(* Logix 5000 AddOnInstructionDefinition export NTEC_READ; software revision ? *)

TYPE NTEC_Axis :   // NTEC Axis:
STRUCT
   StatDriveCommsOK : BOOL;   // Drive is communicating over ENET IP
   StatServoActionStatus : BOOL;   // Motion is enabled and holding position under power.
   StatDriveWarning : BOOL;   // Drive has a Warning
   StatDriveFault : BOOL;   // Drive is Faulted
   StatMotion_AtTarget : BOOL;   // Motion Target Reached
   StatMotion_FollowingError : BOOL;   // Following Error Fault
   StatMotion_LimitExceeded : BOOL;   // Speed or Position Limit Exceeded
   StatMotion_Halt : BOOL;   // Motor is in Halt, still powered on
   StatQuckStop : BOOL;   // Motor is powered off in Quick Stop
   StatMotion_Homed : BOOL;   // Motion Coordinate System Homed
   StatNewCmdToggle : BOOL;   // Bit toggles after new command accepted
   StatCommandError : BOOL;   // Last Command has an Error
   StatCommandErrorCode : DINT;   // Command Error Code
   StatDriveFaultCode : DINT;   // Drive Fault Code
   StatDriveWarningCode : DINT;   // Drive Warning Code
   StatResettingFault : BOOL;   // In fault reset sequence
   StatReadResponse : DINT;   // Response from a Read CMD
   CMD_IP : BOOL;   // Command is In Process
   CMD_DN : BOOL;   // Command is Done
   CMD_ERR : BOOL;   // Command Error during Comms send to Drive
   PDI_CMD : NTEC_PDI_CMD;   // Commands from AOIs
   PDI_Status : NTEC_PDI_Status;   // Status from Drive out to AOIs
   DriveLimits : NTEC_LimitsInDrive;   // Limits read from Drive
END_STRUCT
END_TYPE

TYPE NTEC_LimitsInDrive :   // These are the limits read from the Drive
STRUCT
   PositionLimitMin : DINT;   // Minimum Allowed Position Target (607Bh:1)
   PositionLimitMax : DINT;   // Maximum Allowed Position Target (607Bh:2)
   SoftPositionLimitMin : DINT;   // Minimum Allowed Position (607Dh:1)
   SoftPositionLimitMax : DINT;   // Minimum Allowed Position (607Dh:2)
   VelocityLimitMin : DINT;   // Maximum Allowed Velocity Target negative direction
   VelocityLimitMax : DINT;   // Maximum Allowed Velocity Target positive direction (607Fh)
   MotorSpeedMin : DINT;   // Maximum motor speed in negative direction
   MotorSpeedMax : DINT;   // Maximum motor speed setting in positive direction (6080h)
   AccelLimitMax : DINT;   // Maximum Allowed Accel Target (60C5h)
   DecelLimitMax : DINT;   // Maximum Allowed Decel Target (60C6h)
   PositionWindowNeg : DINT;   // Position Window - negative direction for At Target (6067h)
   PositionWindowPos : DINT;   // Position Window -positive direction for At Target (+/- this value) (6067h)
   VelocityWindowNeg : DINT;   // Velocity Window - negative side for At Target (+/- this value) (606Dh)
   VelocityWindowPos : DINT;   // Velocity Window - positive side for At Target (+/- this value) (606Dh)
   TorqueMaxNegDir : DINT;   // Maximum Torque Target negative direction (0.1% of motor rated current 2031h) (6072h)
   TorqueMaxPosDir : DINT;   // Maximum Torque Target positive direction (0.1% of motor rated current 2031h) (6072h)
   CurrentMaxNegDir : DINT;   // Maximum Current Target negative direction (in 0.1% of rated setting 2031h) (6073h)
   CurrentMaxPosDir : DINT;   // Maximum Current Target positive direction (in 0.1% of rated setting 2031h) (6073h)
END_STRUCT
END_TYPE

TYPE NTEC_PDI_CMD :   // PDI Command Bytes
STRUCT
   SetValue1 : DINT;
   SetValue2 : INT;
   SetValue3 : SINT;
   CMD : SINT;
   DigitalOutputs : DINT;
   NanoJ_Input1 : DINT;
   Trig : BOOL;   // Trigger the Command
   Halt : BOOL;   // Command a HALT
   QuickStop : BOOL;   // Command a QuickStop
END_STRUCT
END_TYPE

TYPE NTEC_PDI_Status :   // PDI Status Bytes
STRUCT
   Status : INT;
   ErrorCode : INT;
   ReturnValue : DINT;
   PositionActualValue : DINT;
   VelocityActualValue : DINT;
   DigitalInputs : DINT;
   TorqueActualValue : INT;
   AnalogInput1 : INT;
   FollowingError : DINT;
   NanoJ_Output1 : DINT;
END_STRUCT
END_TYPE

ADD_ON_INSTRUCTION NTEC_READ   (* revision 1.6, vendor Third Coast Automation, Nashville, TN, ExecutePrescan, ExecuteEnableInFalse *)
// READ instruction reads the value of  one object from the Drive.  Enter the target object's index and sub-index (typically 16#xxxx hex values).
// Revision note:
// Release Aug 27, 2024, update CPS instructions LEN
// Help:
// AOI written by:
// Tim Cochran
// Third Coast Automation
// Nashville, TN
// MAS ERR_Codes:
// 2: Input parameter range error – review and fix input parameters.
// 3: Command Error response from the Drive after command sent.
// 10: Communications Failed to Drive.
// 11: Drive Fault during this AOIs command sequence.
// 12: Quick Stop triggered by software outside of this AOI.
// 13: Command Error response from the Drive.
// 14: Enable input changed to False during sequence due to Drive Fault or Offline.
VAR_IN_OUT
   NTEC_Axis : NTEC_Axis; {required}   // NTEC Axis Tag
END_VAR
VAR_INPUT
   Index : DINT; {required}   // Index
   SubIndex : DINT; {required}   // Sub-Index
END_VAR
VAR_OUTPUT
   EN : BOOL; {visible}   // Enabled
   DN : BOOL; {visible}   // Successfully Done
   Read_Value : DINT; {visible}   // Value Read from Drive
   ERR : BOOL; {visible}   // Instruction Error
   ERR_Code : DINT; {access Read Only, visible}   // Instruction Error Code
END_VAR
VAR
   State : DINT; {access None}
   Enable : BOOL; {access None}
   InputRangesOK : BOOL; {access None}
   local_SubIndex : DINT; {access None}
   local_Index : DINT; {access None}
   tmr_Verify : TIMER := (PRE := 20); {access None}
END_VAR

ROUTINE EnableInFalse   (* ladder *)
// Enable In False Routine
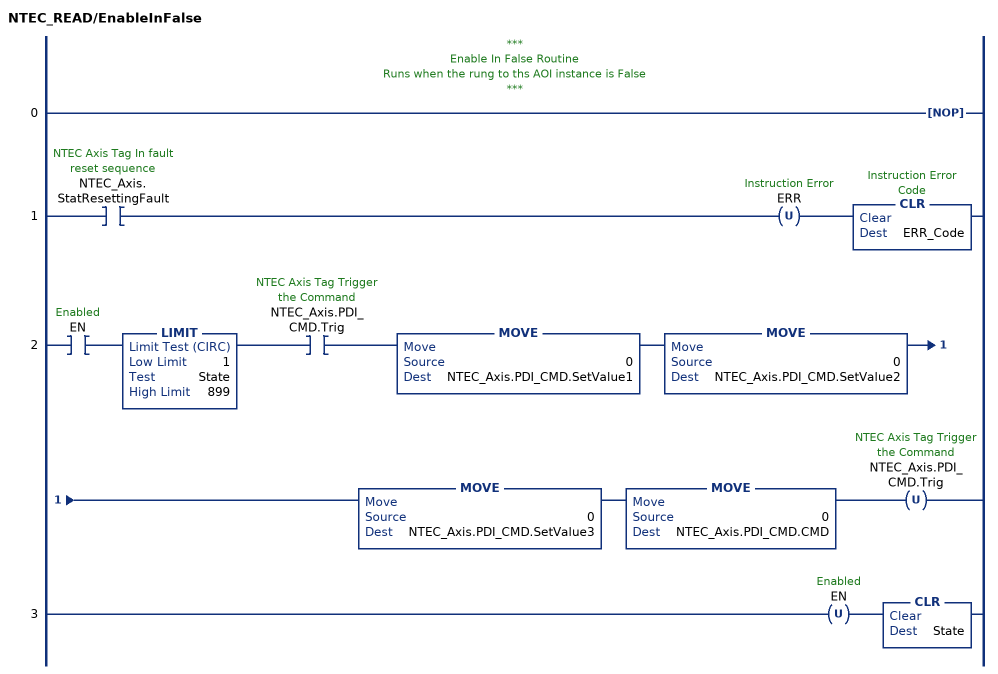
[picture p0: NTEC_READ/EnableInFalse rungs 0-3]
   // ***
   // Enable In False Routine
   // Runs when the rung to ths AOI instance is False
   // ***
   0: NOP();
   1: XIC(NTEC_Axis.StatResettingFault)OTU(ERR)CLR(ERR_Code);
   2: XIC(EN)LIMIT(1,State,899)XIC(NTEC_Axis.PDI_CMD.Trig)MOVE(0,NTEC_Axis.PDI_CMD.SetValue1)MOVE(0,NTEC_Axis.PDI_CMD.SetValue2)MOVE(0,NTEC_Axis.PDI_CMD.SetValue3)MOVE(0,NTEC_Axis.PDI_CMD.CMD)OTU(NTEC_Axis.PDI_CMD.Trig);
   3: OTU(EN)CLR(State);
END_ROUTINE

ROUTINE Logic   (* ladder *)
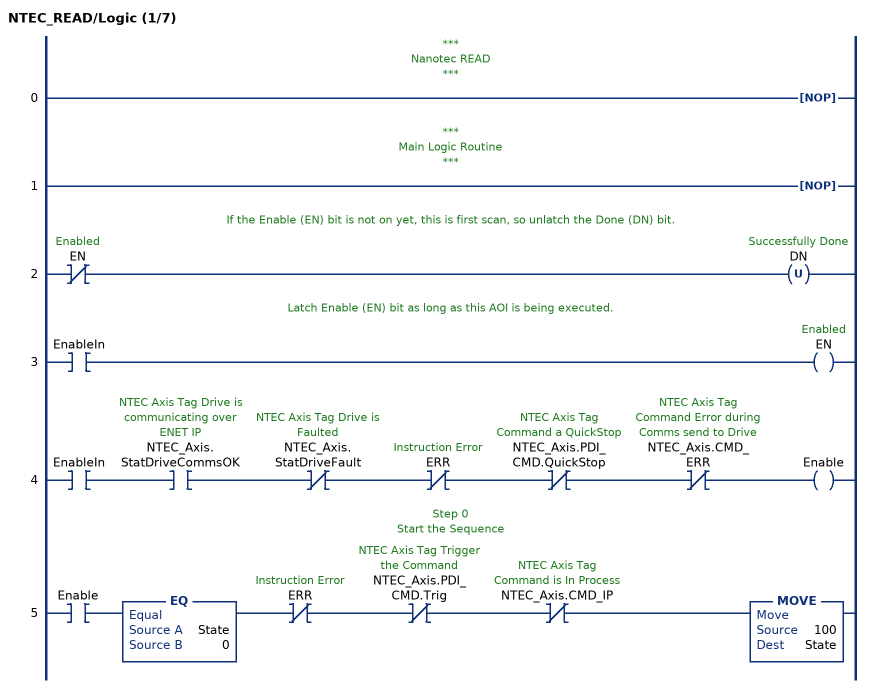
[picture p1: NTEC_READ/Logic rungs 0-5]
   // ***
   // Nanotec READ
   // ***
   0: NOP();
   // ***
   // Main Logic Routine
   // ***
   1: NOP();
   // If the Enable (EN) bit is not on yet, this is first scan, so unlatch the Done (DN) bit.
   2: XIO(EN)OTU(DN);
   // Latch Enable (EN) bit as long as this AOI is being executed.
   3: XIC(EnableIn)OTE(EN);
   4: XIC(EnableIn)XIC(NTEC_Axis.StatDriveCommsOK)XIO(NTEC_Axis.StatDriveFault)XIO(ERR)XIO(NTEC_Axis.PDI_CMD.QuickStop)XIO(NTEC_Axis.CMD_ERR)OTE(Enable);
   // Step 0
   // Start the Sequence
   5: XIC(Enable)EQ(State,0)XIO(ERR)XIO(NTEC_Axis.PDI_CMD.Trig)XIO(NTEC_Axis.CMD_IP)MOVE(100,State);
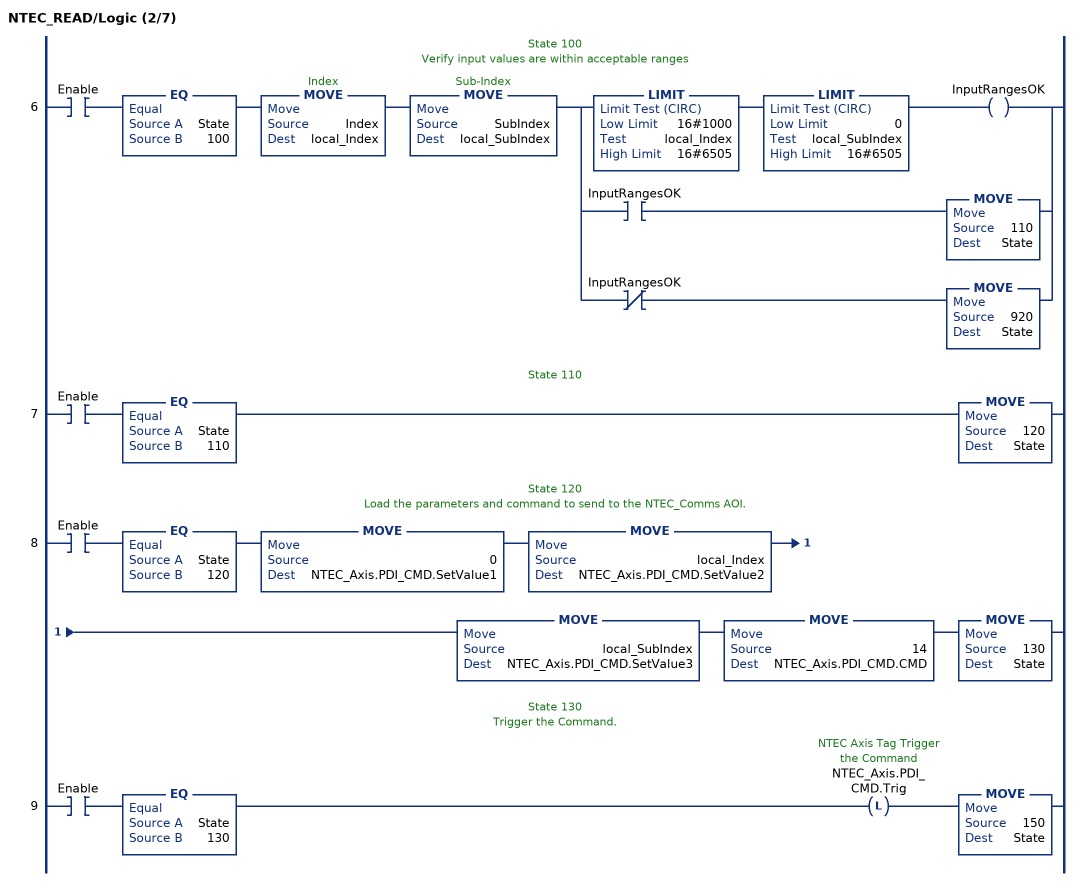
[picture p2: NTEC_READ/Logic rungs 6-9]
   // State 100
   // Verify input values are within acceptable ranges
   6: XIC(Enable)EQ(State,100)MOVE(Index,local_Index)MOVE(SubIndex,local_SubIndex)[LIMIT(16#1000,local_Index,16#6505) LIMIT(0,local_SubIndex,16#6505) OTE(InputRangesOK) ,XIC(InputRangesOK) MOVE(110,State) ,XIO(InputRangesOK) MOVE(920,State) ];
   // State 110
   7: XIC(Enable)EQ(State,110)MOVE(120,State);
   // State 120
   // Load the parameters and command to send to the NTEC_Comms AOI.
   8: XIC(Enable)EQ(State,120)MOVE(0,NTEC_Axis.PDI_CMD.SetValue1)MOVE(local_Index,NTEC_Axis.PDI_CMD.SetValue2)MOVE(local_SubIndex,NTEC_Axis.PDI_CMD.SetValue3)MOVE(14,NTEC_Axis.PDI_CMD.CMD)MOVE(130,State);
   // State 130
   // Trigger the Command.
   9: XIC(Enable)EQ(State,130)OTL(NTEC_Axis.PDI_CMD.Trig)MOVE(150,State);
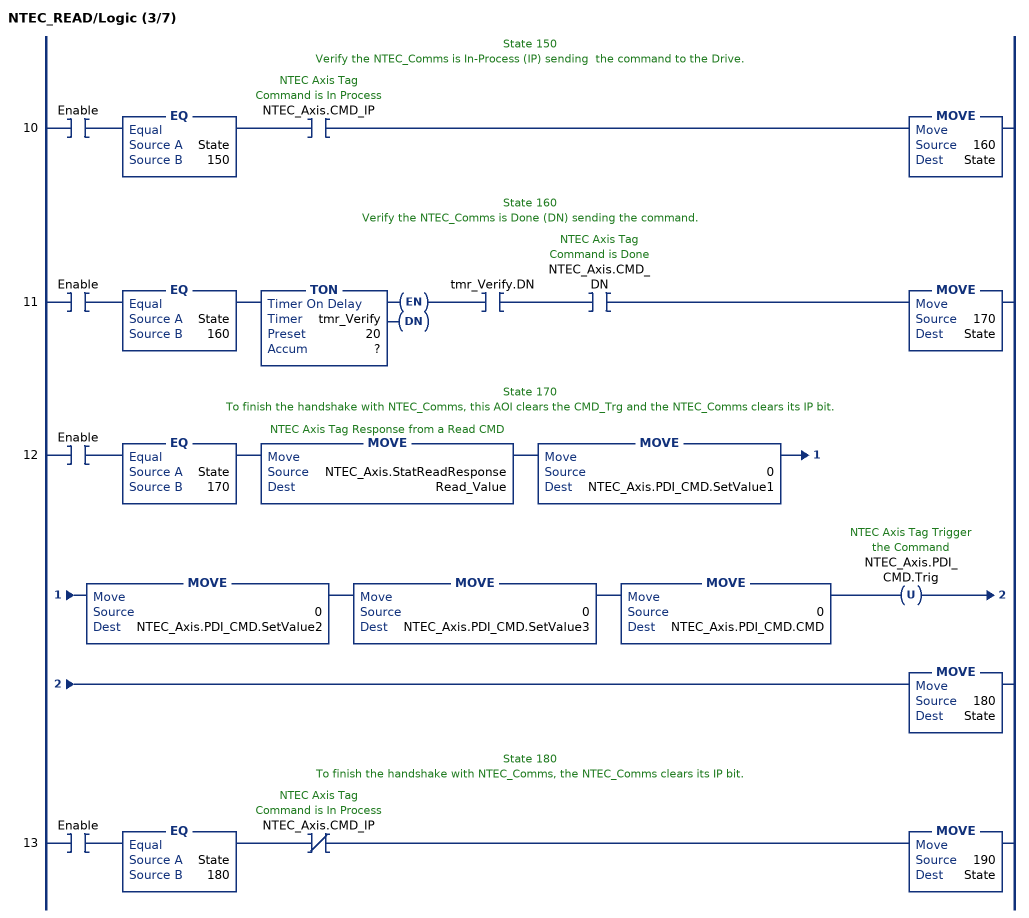
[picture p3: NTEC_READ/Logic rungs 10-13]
   // State 150
   // Verify the NTEC_Comms is In-Process (IP) sending  the command to the Drive.
   10: XIC(Enable)EQ(State,150)XIC(NTEC_Axis.CMD_IP)MOVE(160,State);
   // State 160
   // Verify the NTEC_Comms is Done (DN) sending the command.
   11: XIC(Enable)EQ(State,160)TON(tmr_Verify,?,?)XIC(tmr_Verify.DN)XIC(NTEC_Axis.CMD_DN)MOVE(170,State);
   // State 170
   // To finish the handshake with NTEC_Comms, this AOI clears the CMD_Trg and the NTEC_Comms clears its IP bit.
   12: XIC(Enable)EQ(State,170)MOVE(NTEC_Axis.StatReadResponse,Read_Value)MOVE(0,NTEC_Axis.PDI_CMD.SetValue1)MOVE(0,NTEC_Axis.PDI_CMD.SetValue2)MOVE(0,NTEC_Axis.PDI_CMD.SetValue3)MOVE(0,NTEC_Axis.PDI_CMD.CMD)OTU(NTEC_Axis.PDI_CMD.Trig)MOVE(180,State);
   // State 180
   // To finish the handshake with NTEC_Comms, the NTEC_Comms clears its IP bit.
   13: XIC(Enable)EQ(State,180)XIO(NTEC_Axis.CMD_IP)MOVE(190,State);
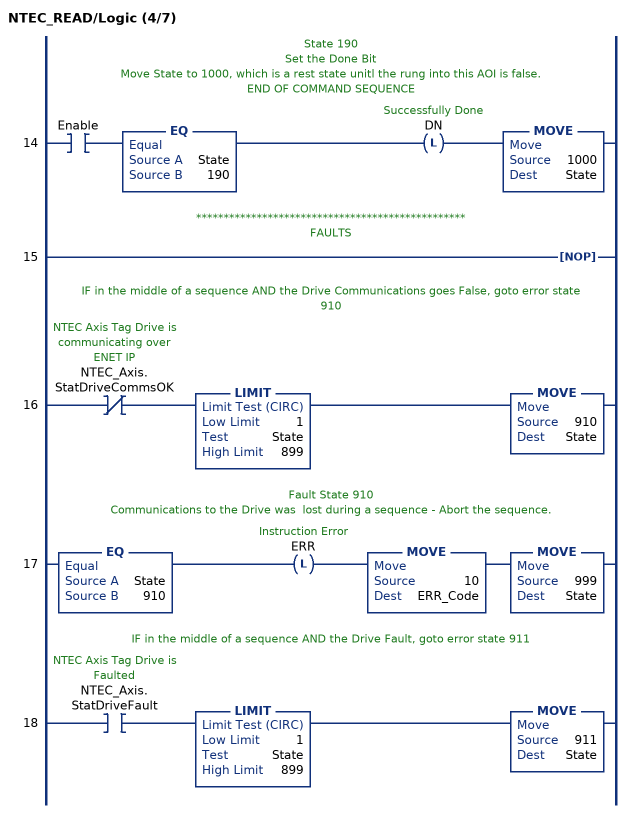
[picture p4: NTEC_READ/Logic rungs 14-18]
   // State 190
   // Set the Done Bit
   // Move State to 1000, which is a rest state unitl the rung into this AOI is false.
   // END OF COMMAND SEQUENCE
   14: XIC(Enable)EQ(State,190)OTL(DN)MOVE(1000,State);
   // *************************************************
   // FAULTS
   15: NOP();
   // IF in the middle of a sequence AND the Drive Communications goes False, goto error state 910
   16: XIO(NTEC_Axis.StatDriveCommsOK)LIMIT(1,State,899)MOVE(910,State);
   // Fault State 910
   // Communications to the Drive was  lost during a sequence - Abort the sequence.
   17: EQ(State,910)OTL(ERR)MOVE(10,ERR_Code)MOVE(999,State);
   // IF in the middle of a sequence AND the Drive Fault, goto error state 911
   18: XIC(NTEC_Axis.StatDriveFault)LIMIT(1,State,899)MOVE(911,State);
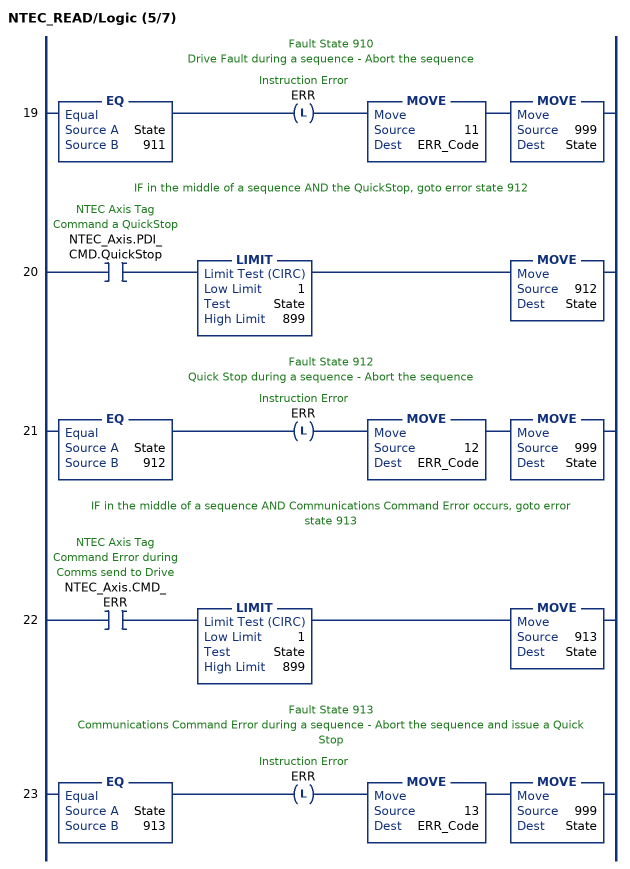
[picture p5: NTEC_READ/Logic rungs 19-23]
   // Fault State 910
   // Drive Fault during a sequence - Abort the sequence
   19: EQ(State,911)OTL(ERR)MOVE(11,ERR_Code)MOVE(999,State);
   // IF in the middle of a sequence AND the QuickStop, goto error state 912
   20: XIC(NTEC_Axis.PDI_CMD.QuickStop)LIMIT(1,State,899)MOVE(912,State);
   // Fault State 912
   // Quick Stop during a sequence - Abort the sequence
   21: EQ(State,912)OTL(ERR)MOVE(12,ERR_Code)MOVE(999,State);
   // IF in the middle of a sequence AND Communications Command Error occurs, goto error state 913
   22: XIC(NTEC_Axis.CMD_ERR)LIMIT(1,State,899)MOVE(913,State);
   // Fault State 913
   // Communications Command Error during a sequence - Abort the sequence and issue a Quick Stop
   23: EQ(State,913)OTL(ERR)MOVE(13,ERR_Code)MOVE(999,State);
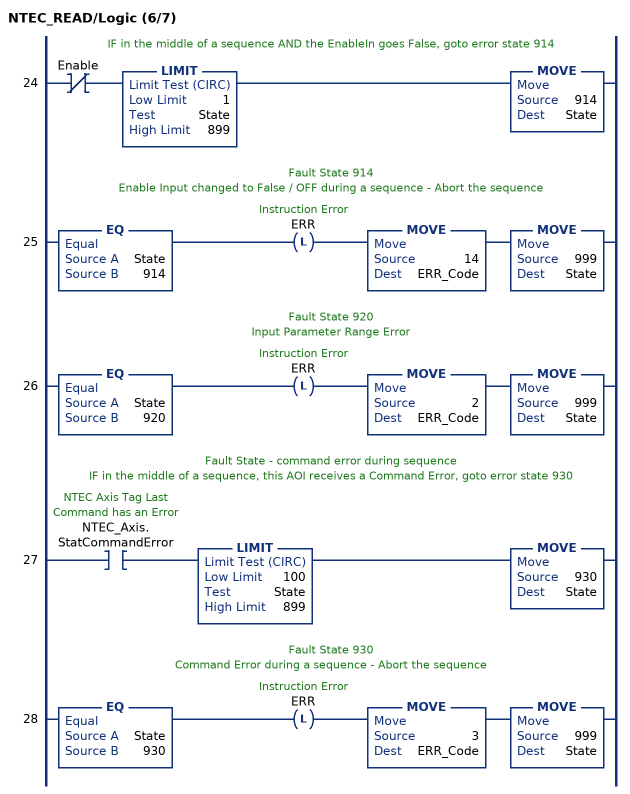
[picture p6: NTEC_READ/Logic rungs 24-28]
   // IF in the middle of a sequence AND the EnableIn goes False, goto error state 914
   24: XIO(Enable)LIMIT(1,State,899)MOVE(914,State);
   // Fault State 914
   // Enable Input changed to False / OFF during a sequence - Abort the sequence
   25: EQ(State,914)OTL(ERR)MOVE(14,ERR_Code)MOVE(999,State);
   // Fault State 920
   // Input Parameter Range Error
   26: EQ(State,920)OTL(ERR)MOVE(2,ERR_Code)MOVE(999,State);
   // Fault State - command error during sequence
   // IF in the middle of a sequence, this AOI receives a Command Error, goto error state 930
   27: XIC(NTEC_Axis.StatCommandError)LIMIT(100,State,899)MOVE(930,State);
   // Fault State 930
   // Command Error during a sequence - Abort the sequence
   28: EQ(State,930)OTL(ERR)MOVE(3,ERR_Code)MOVE(999,State);
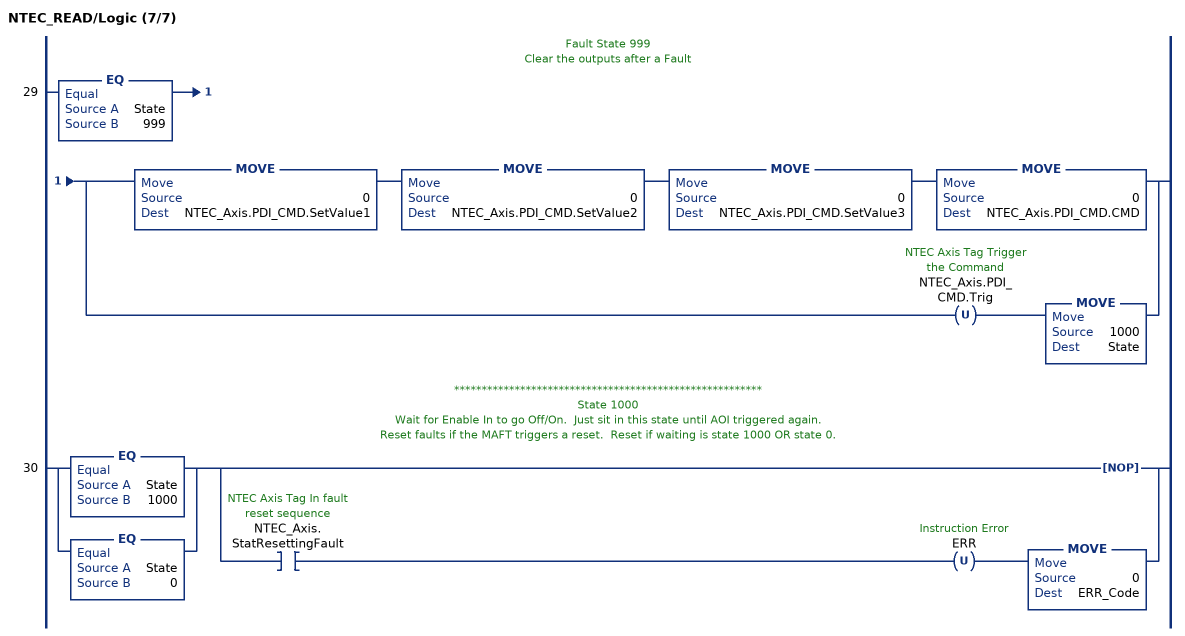
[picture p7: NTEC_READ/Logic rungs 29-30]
   // Fault State 999
   // Clear the outputs after a Fault
   29: EQ(State,999)[MOVE(0,NTEC_Axis.PDI_CMD.SetValue1) MOVE(0,NTEC_Axis.PDI_CMD.SetValue2) MOVE(0,NTEC_Axis.PDI_CMD.SetValue3) MOVE(0,NTEC_Axis.PDI_CMD.CMD) ,OTU(NTEC_Axis.PDI_CMD.Trig) MOVE(1000,State) ];
   // ********************************************************
   // State 1000
   // Wait for Enable In to go Off/On.  Just sit in this state until AOI triggered again.
   // Reset faults if the MAFT triggers a reset.  Reset if waiting is state 1000 OR state 0.
   30: [EQ(State,1000) ,EQ(State,0) ][NOP() ,XIC(NTEC_Axis.StatResettingFault) OTU(ERR) MOVE(0,ERR_Code) ];
END_ROUTINE

ROUTINE Postscan   (* ladder *)
// Home Post-Scan Routine
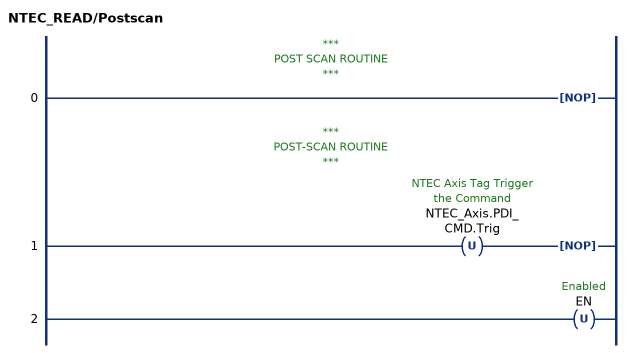
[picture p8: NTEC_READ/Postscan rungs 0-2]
   // ***
   // POST SCAN ROUTINE
   // ***
   0: NOP();
   // ***
   // POST-SCAN ROUTINE
   // ***
   1: OTU(NTEC_Axis.PDI_CMD.Trig)NOP();
   2: OTU(EN);
END_ROUTINE

ROUTINE Prescan   (* ladder *)
// Home Pre-Scan Routine
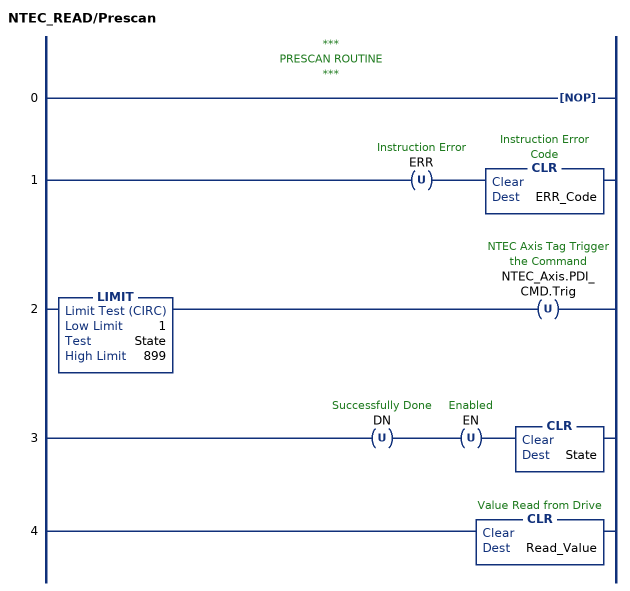
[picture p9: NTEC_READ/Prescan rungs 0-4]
   // ***
   // PRESCAN ROUTINE
   // ***
   0: NOP();
   1: OTU(ERR)CLR(ERR_Code);
   2: LIMIT(1,State,899)OTU(NTEC_Axis.PDI_CMD.Trig);
   3: OTU(DN)OTU(EN)CLR(State);
   4: CLR(Read_Value);
END_ROUTINE
END_ADD_ON_INSTRUCTION
